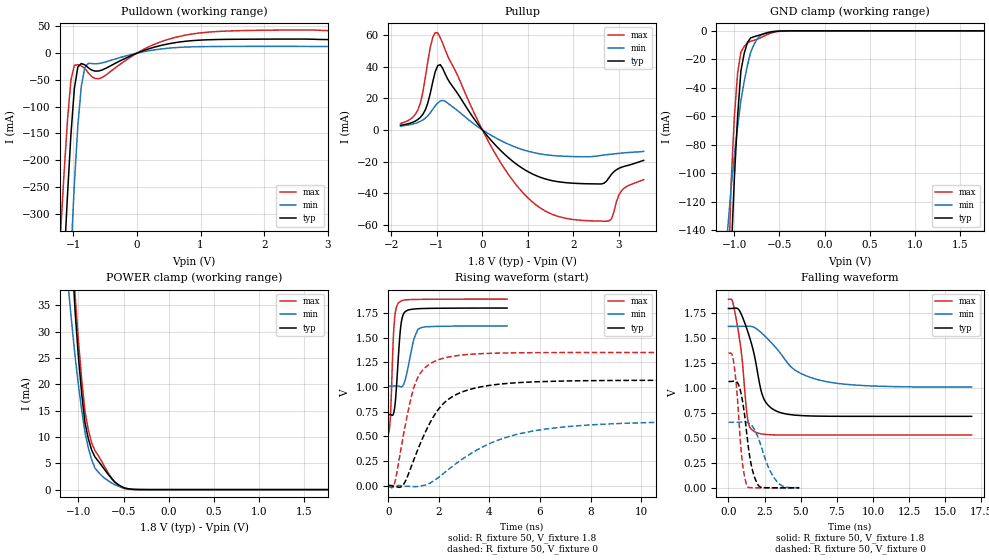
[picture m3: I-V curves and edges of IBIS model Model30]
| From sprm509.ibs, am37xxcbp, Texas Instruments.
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| Model based on original model for BQ18OMAPSMART1HYFBPBNOPM_SSBHH
|   Sub model PM_HS10L11_PUPD0_1P8
[model]   Model30
|[Input Load]   PI
|[Output Drive] SC10LB11
|Voltage   1.8V
|Mode   I/O
Model_type   I/O
Polarity   Non-Inverting
Enable   Active-Low
Vinl =  0.63
Vinh =  1.17
Cref =  15pF
Rref =  100.0000M
Vref =  0V
Vmeas =  0.9
C_comp   1.410688p   1.256095p   1.577871p
[Model Spec]
Vinl   0.63   0.567   0.6615
Vinh   1.17   1.053   1.2285
[Temperature Range]   25   125   -40
[Voltage Range]   1.8   1.62   1.89
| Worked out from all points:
|   slope of the pulldown table from 0 to 0.27 V, typ, clamps not added: 24.3 ohm
|   slope of the pullup table from 0 to 0.27 V, typ, clamps not added: 29.7 ohm
|   GND clamp passes 1 mA (typ) near -0.60 V on its own axis
|   POWER clamp passes 1 mA (typ) near -0.56 V on its own axis
|   rising waveform, R_fixture 50, V_fixture 1.8: 20-80 % time 176ps typ, 302ps min, 124ps max; typ from 0.718 V to 1.8 V
|   rising waveform, R_fixture 50, V_fixture 0: 20-80 % time 1.34ns typ, 2.95ns min, 707ps max; typ from 0 V to 1.07 V
|   falling waveform, R_fixture 50, V_fixture 1.8: 20-80 % time 1.04ns typ, 2.54ns min, 608ps max; typ from 1.8 V to 0.718 V
|   falling waveform, R_fixture 50, V_fixture 0: 20-80 % time 611ps typ, 1.03ns min, 438ps max; typ from 1.07 V to 0 V
[POWER_clamp]
-1.8V     362.5mA    191.4mA    412.8mA
-1.109V   56.69mA    37.71mA    60.38mA
-1.073V   44.6mA     31.22mA    47.8mA
-1.036V   33.44mA    25.04mA    36.59mA
-1V       24.98mA    19.72mA    28.06mA
-963.6mV  18.03mA    14.96mA    20.78mA
-927.3mV  12.59mA    10.77mA    14.74mA
-890.9mV  9.653mA    7.899mA    11.31mA
-818.2mV  6.214mA    4.114mA    7.414mA
-636.4mV  2.183mA    1.307mA    2.238mA
-418.2mV  83.85uA    105.2uA    35.14uA
1.764V    -1.228nA   -79.12nA   -1.453nA
[Pulldown]
-1.8V     -1.718A    -2.61A     -1.406A
-1.2V     -527.4mA   -844.5mA   -339.9mA
-1.145V   -396mA     -683.1mA   -229.1mA
-1.091V   -269mA     -526.7mA   -127.5mA
-1.036V   -153.6mA   -378.9mA   -51.17mA
-981.8mV  -66.34mA   -245.6mA   -22.67mA
-927.3mV  -26mA      -136.2mA   -21.54mA
-872.7mV  -19.34mA   -61.98mA   -23.69mA
-763.6mV  -27.2mA    -19.05mA   -36.72mA
-545.5mV  -31.39mA   -18.17mA   -45.46mA
872.7mV   23.46mA    11.88mA    35.92mA
3.545V    25.34mA    12.51mA    41.58mA
[Pullup]
-1.8V     2.903mA    2.423mA    4.112mA
-1.418V   6.595mA    4.711mA    12.64mA
-1.255V   12.69mA    7.42mA     33.23mA
-1.091V   30.4mA     13mA       58.69mA
-981.8mV  40.63mA    17.02mA    61.3mA
-818.2mV  35.38mA    18.12mA    50.59mA
272.7mV   -9.18mA    -4.728mA   -14.55mA
1.255V    -29.75mA   -15.09mA   -48.97mA
2.564V    -34.17mA   -16.31mA   -57.57mA
2.782V    -30.25mA   -15.5mA    -57.48mA
3.055V    -23.63mA   -14.68mA   -38.61mA
3.545V    -19.25mA   -13.56mA   -31.41mA
[GND_clamp]
-1.8V     -2.82A     -1.192A    -3.165A
-1.073V   -235.7mA   -138.4mA   -192.1mA
-1.036V   -159.5mA   -110.8mA   -107.5mA
-1V       -103.8mA   -87.85mA   -60.67mA
-963.6mV  -60mA      -67.28mA   -29.8mA
-927.3mV  -28.21mA   -49.08mA   -14.9mA
-890.9mV  -15.9mA    -35.48mA   -10.99mA
-854.5mV  -8.138mA   -24.07mA   -8.449mA
-818.2mV  -4.924mA   -14.85mA   -7.266mA
-709.1mV  -2.784mA   -3.064mA   -4.883mA
-563.6mV  -570.2uA   -404.5uA   -1.092mA
1.764V    -11.02pA   583.5nA    3.035nA
[Ramp]
dV/dt_f  0.6514011/1.04235n   0.3678968/2.564283n   0.8183331/0.6102358n
dV/dt_r  0.6512504/1.344153n   0.4008455/2.976144n   0.82315/0.7085103n
R_load = 50
[Rising Waveform]
R_fixture = 50
V_fixture = 1.8
V_fixture_min = 1.62
V_fixture_max = 1.89
0s        717.6mV    1.009V     527.1mV
81ps      719.5mV    1.009V     697.5mV
180ps     715.9mV    1.009V     1.395V
225ps     751.3mV    1.01V      1.625V
288ps     886.8mV    1.011V     1.772V
396ps     1.305V     1.01V      1.85V
495ps     1.624V     1V         1.869V
576ps     1.726V     1.013V     1.878V
1.17ns    1.793V     1.584V     1.887V
4.698ns   1.799V     1.618V     1.89V
[Rising Waveform]
R_fixture = 50
V_fixture = 0
V_fixture_min = 0
V_fixture_max = 0
0s        162.4uV    77.16uV    -10.13mV
234ps     -9.518mV   -48.66uV   11.76mV
612ps     16.44mV    -4.257mV   533.6mV
891ps     182.6mV    -8.609mV   881.6mV
1.125ns   339.2mV    -9.701mV   1.074V
1.692ns   657.7mV    31.71mV    1.24V
2.205ns   837.7mV    128mV      1.293V
4.149ns   1.021V     441.2mV    1.341V
6.417ns   1.056V     579.6mV    1.348V
20.24ns   1.067V     655.8mV    1.349V
[Falling Waveform]
R_fixture = 50
V_fixture = 1.8
V_fixture_min = 1.62
V_fixture_max = 1.89
0s        1.8V       1.62V      1.89V
306ps     1.801V     1.62V      1.859V
711ps     1.789V     1.62V      1.547V
1.386ns   1.546V     1.622V     645.2mV
1.827ns   1.306V     1.606V     562.8mV
2.466ns   887.2mV    1.531V     537.5mV
3.627ns   753.8mV    1.344V     530.5mV
4.797ns   727.8mV    1.164V     529.9mV
7.155ns   718.4mV    1.056V     529.8mV
16.82ns   717.6mV    1.011V     529.8mV
[Falling Waveform]
R_fixture = 50
V_fixture = 0
V_fixture_min = 0
V_fixture_max = 0
0s        1.067V     657.3mV    1.349V
360ps     1.071V     657.3mV    1.262V
594ps     1.06V      657.5mV    952.4mV
945ps     894.2mV    660.7mV    277.7mV
1.305ns   497.2mV    655.8mV    14.68mV
1.665ns   175.8mV    615.8mV    1.554mV
2.088ns   21.72mV    491.4mV    271.4uV
2.727ns   1.478mV    220.9mV    30.09uV
3.33ns    396.9uV    68.57mV    6.356uV
4.896ns   58.63uV    1.629mV    604.9nV
